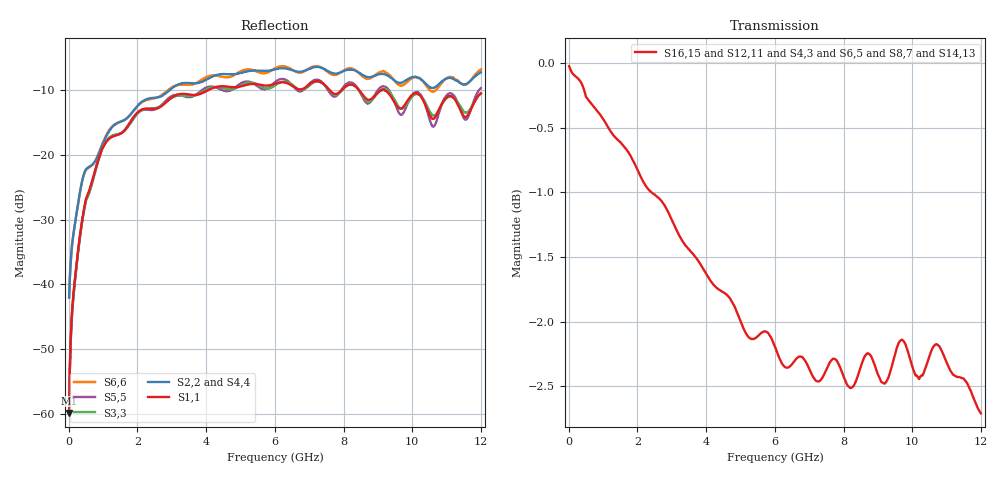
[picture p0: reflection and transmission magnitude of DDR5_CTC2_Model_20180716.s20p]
! Created Mon Jul 16 16:07:11 2018
! Port 1 = DQ8 SMP
! Port 2 = DQ8 DIMM+2.7mm
! Port 3 = DQ9 SMP
! Port 4 = DQ9 DIMM+2.7mm
! Port 5 = DQ10 SMP
! Port 6 = DQ10 DIMM+2.7mm
! Port 7 = DQ11 SMP
! Port 8 = DQ11 DIMM+2.7mm
! Port 9 = DQ12 SMP
! Port 10 = DQ12 DIMM+2.7mm
! Port 11 = DQ13 SMP
! Port 12 = DQ13 DIMM+2.7mm
! Port 13 = DQ14 SMP
! Port 14 = DQ14 DIMM+2.7mm
! Port 15 = DQ15 SMP
! Port 16 = DQ15 DIMM+2.7mm
! Port 17 = DQS_t SMP
! Port 18 = DQS_t DIMM+2.7mm
! Port 19 = DQS_c SMP
! Port 20 = DQS_c DIMM+2.7mm
! 20 Port Network Data from SP1.SP block
! freq  magS1_1  angS1_1  magS1_2  angS1_2  magS1_3  angS1_3  magS1_4  angS1_4
!  magS1_5  angS1_5  magS1_6  angS1_6  magS1_7  angS1_7  magS1_8  angS1_8
!  magS1_9  angS1_9  magS1_10  angS1_10  magS1_11  angS1_11  magS1_12  angS1_12
!  magS1_13  angS1_13  magS1_14  angS1_14  magS1_15  angS1_15  magS1_16  angS1_16
!  magS1_17  angS1_17  magS1_18  angS1_18  magS1_19  angS1_19  magS1_20  angS1_20
!  magS2_1  angS2_1  magS2_2  angS2_2  magS2_3  angS2_3  magS2_4  angS2_4
!  magS2_5  angS2_5  magS2_6  angS2_6  magS2_7  angS2_7  magS2_8  angS2_8
!  magS2_9  angS2_9  magS2_10  angS2_10  magS2_11  angS2_11  magS2_12  angS2_12
!  magS2_13  angS2_13  magS2_14  angS2_14  magS2_15  angS2_15  magS2_16  angS2_16
!  magS2_17  angS2_17  magS2_18  angS2_18  magS2_19  angS2_19  magS2_20  angS2_20
!  magS3_1  angS3_1  magS3_2  angS3_2  magS3_3  angS3_3  magS3_4  angS3_4
!  magS3_5  angS3_5  magS3_6  angS3_6  magS3_7  angS3_7  magS3_8  angS3_8
!  magS3_9  angS3_9  magS3_10  angS3_10  magS3_11  angS3_11  magS3_12  angS3_12
!  magS3_13  angS3_13  magS3_14  angS3_14  magS3_15  angS3_15  magS3_16  angS3_16
!  magS3_17  angS3_17  magS3_18  angS3_18  magS3_19  angS3_19  magS3_20  angS3_20
!  magS4_1  angS4_1  magS4_2  angS4_2  magS4_3  angS4_3  magS4_4  angS4_4
!  magS4_5  angS4_5  magS4_6  angS4_6  magS4_7  angS4_7  magS4_8  angS4_8
!  magS4_9  angS4_9  magS4_10  angS4_10  magS4_11  angS4_11  magS4_12  angS4_12
!  magS4_13  angS4_13  magS4_14  angS4_14  magS4_15  angS4_15  magS4_16  angS4_16
!  magS4_17  angS4_17  magS4_18  angS4_18  magS4_19  angS4_19  magS4_20  angS4_20
!  magS5_1  angS5_1  magS5_2  angS5_2  magS5_3  angS5_3  magS5_4  angS5_4
!  magS5_5  angS5_5  magS5_6  angS5_6  magS5_7  angS5_7  magS5_8  angS5_8
!  magS5_9  angS5_9  magS5_10  angS5_10  magS5_11  angS5_11  magS5_12  angS5_12
!  magS5_13  angS5_13  magS5_14  angS5_14  magS5_15  angS5_15  magS5_16  angS5_16
!  magS5_17  angS5_17  magS5_18  angS5_18  magS5_19  angS5_19  magS5_20  angS5_20
!  magS6_1  angS6_1  magS6_2  angS6_2  magS6_3  angS6_3  magS6_4  angS6_4
!  magS6_5  angS6_5  magS6_6  angS6_6  magS6_7  angS6_7  magS6_8  angS6_8
!  magS6_9  angS6_9  magS6_10  angS6_10  magS6_11  angS6_11  magS6_12  angS6_12
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# hz S ma R 50
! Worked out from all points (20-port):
!   1200 points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, 10 MHz to 12 GHz, reference 50 ohm
!   strongest paths, dB at 10 MHz, 3.01 GHz, 6.01 GHz, 9.01 GHz, 12 GHz:
!     S16,15: 0.0, -1.2, -2.2, -2.4, -2.7
!     S12,11: 0.0, -1.2, -2.3, -2.4, -2.9
!     S4,3: 0.0, -1.2, -2.2, -2.4, -2.9
!     S6,5: 0.0, -1.3, -2.2, -2.4, -3.0
!     S8,7: 0.0, -1.3, -2.2, -2.4, -2.9
!     S14,13: 0.0, -1.2, -2.2, -2.4, -2.9
!   lowest |S11| = -59.9 dB at 10 MHz (marker M1), VSWR 1.00, Z = 49.9 + j0.0524 ohm
!   |S11| at or under -10 dB: start of sweep to 4.052 GHz; 8.458 GHz to 9.116 GHz (658.6 MHz wide, 7.49 % of centre); 9.192 GHz to end of sweep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
